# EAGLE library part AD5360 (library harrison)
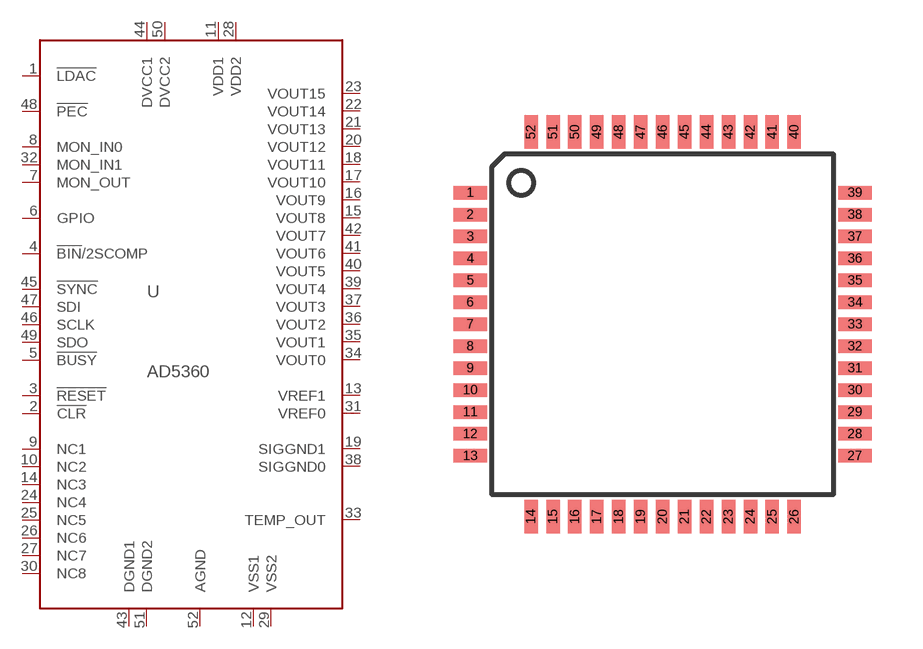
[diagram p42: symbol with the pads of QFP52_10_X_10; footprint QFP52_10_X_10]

Designator prefix U

## AD5360-QFP  [QFP52_10_X_10]
1  !LDAC!  in
2  !CLR!  in
3  !RESET!  in
4  !BIN!/2SCOMP  in
5  !BUSY!
6  GPIO
7  MON_OUT  out
8  MON_IN0  in
9  NC1  nc
10  NC2  nc
11  VDD1  pwr
12  VSS1  pwr
13  VREF1  in
14  NC3  nc
15  VOUT8  out
16  VOUT9  out
17  VOUT10  out
18  VOUT11  out
19  SIGGND1  pwr
20  VOUT12  out
21  VOUT13  out
22  VOUT14  out
23  VOUT15  out
24  NC4  nc
25  NC5  nc
26  NC6  nc
27  NC7  nc
28  VDD2  pwr
29  VSS2  pwr
30  NC8  nc
31  VREF0  in
32  MON_IN1  in
33  TEMP_OUT  out
34  VOUT0  out
35  VOUT1  out
36  VOUT2  out
37  VOUT3  out
38  SIGGND0  pwr
39  VOUT4  out
40  VOUT5  out
41  VOUT6  out
42  VOUT7  out
43  DGND1  pwr
44  DVCC1  pwr
45  !SYNC!  in
46  SCLK  in
47  SDI  in
48  !PEC!  out
49  SDO  out
50  DVCC2  pwr
51  DGND2  pwr
52  AGND  pwr

## Footprint QFP52_10_X_10 (pad centres in mm)
smd 1 x 0.4: 1 -5.7,3.9; 2 -5.7,3.25; 3 -5.7,2.6; 4 -5.7,1.95; 5 -5.7,1.3; 6 -5.7,0.65; 7 -5.7,0; 8 -5.7,-0.65; 9 -5.7,-1.3; 10 -5.7,-1.95; 11 -5.7,-2.6; 12 -5.7,-3.25; 13 -5.7,-3.9; 27 5.7,-3.9; 28 5.7,-3.25; 29 5.7,-2.6; 30 5.7,-1.95; 31 5.7,-1.3; 32 5.7,-0.65; 33 5.7,0; 34 5.7,0.65; 35 5.7,1.3; 36 5.7,1.95; 37 5.7,2.6; 38 5.7,3.25; 39 5.7,3.9
smd 0.4 x 1: 14 -3.9,-5.7; 15 -3.25,-5.7; 16 -2.6,-5.7; 17 -1.95,-5.7; 18 -1.3,-5.7; 19 -0.65,-5.7; 20 0,-5.7; 21 0.65,-5.7; 22 1.3,-5.7; 23 1.95,-5.7; 24 2.6,-5.7; 25 3.25,-5.7; 26 3.9,-5.7; 40 3.9,5.7; 41 3.25,5.7; 42 2.6,5.7; 43 1.95,5.7; 44 1.3,5.7; 45 0.65,5.7; 46 0,5.7; 47 -0.65,5.7; 48 -1.3,5.7; 49 -1.95,5.7; 50 -2.6,5.7; 51 -3.25,5.7; 52 -3.9,5.7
